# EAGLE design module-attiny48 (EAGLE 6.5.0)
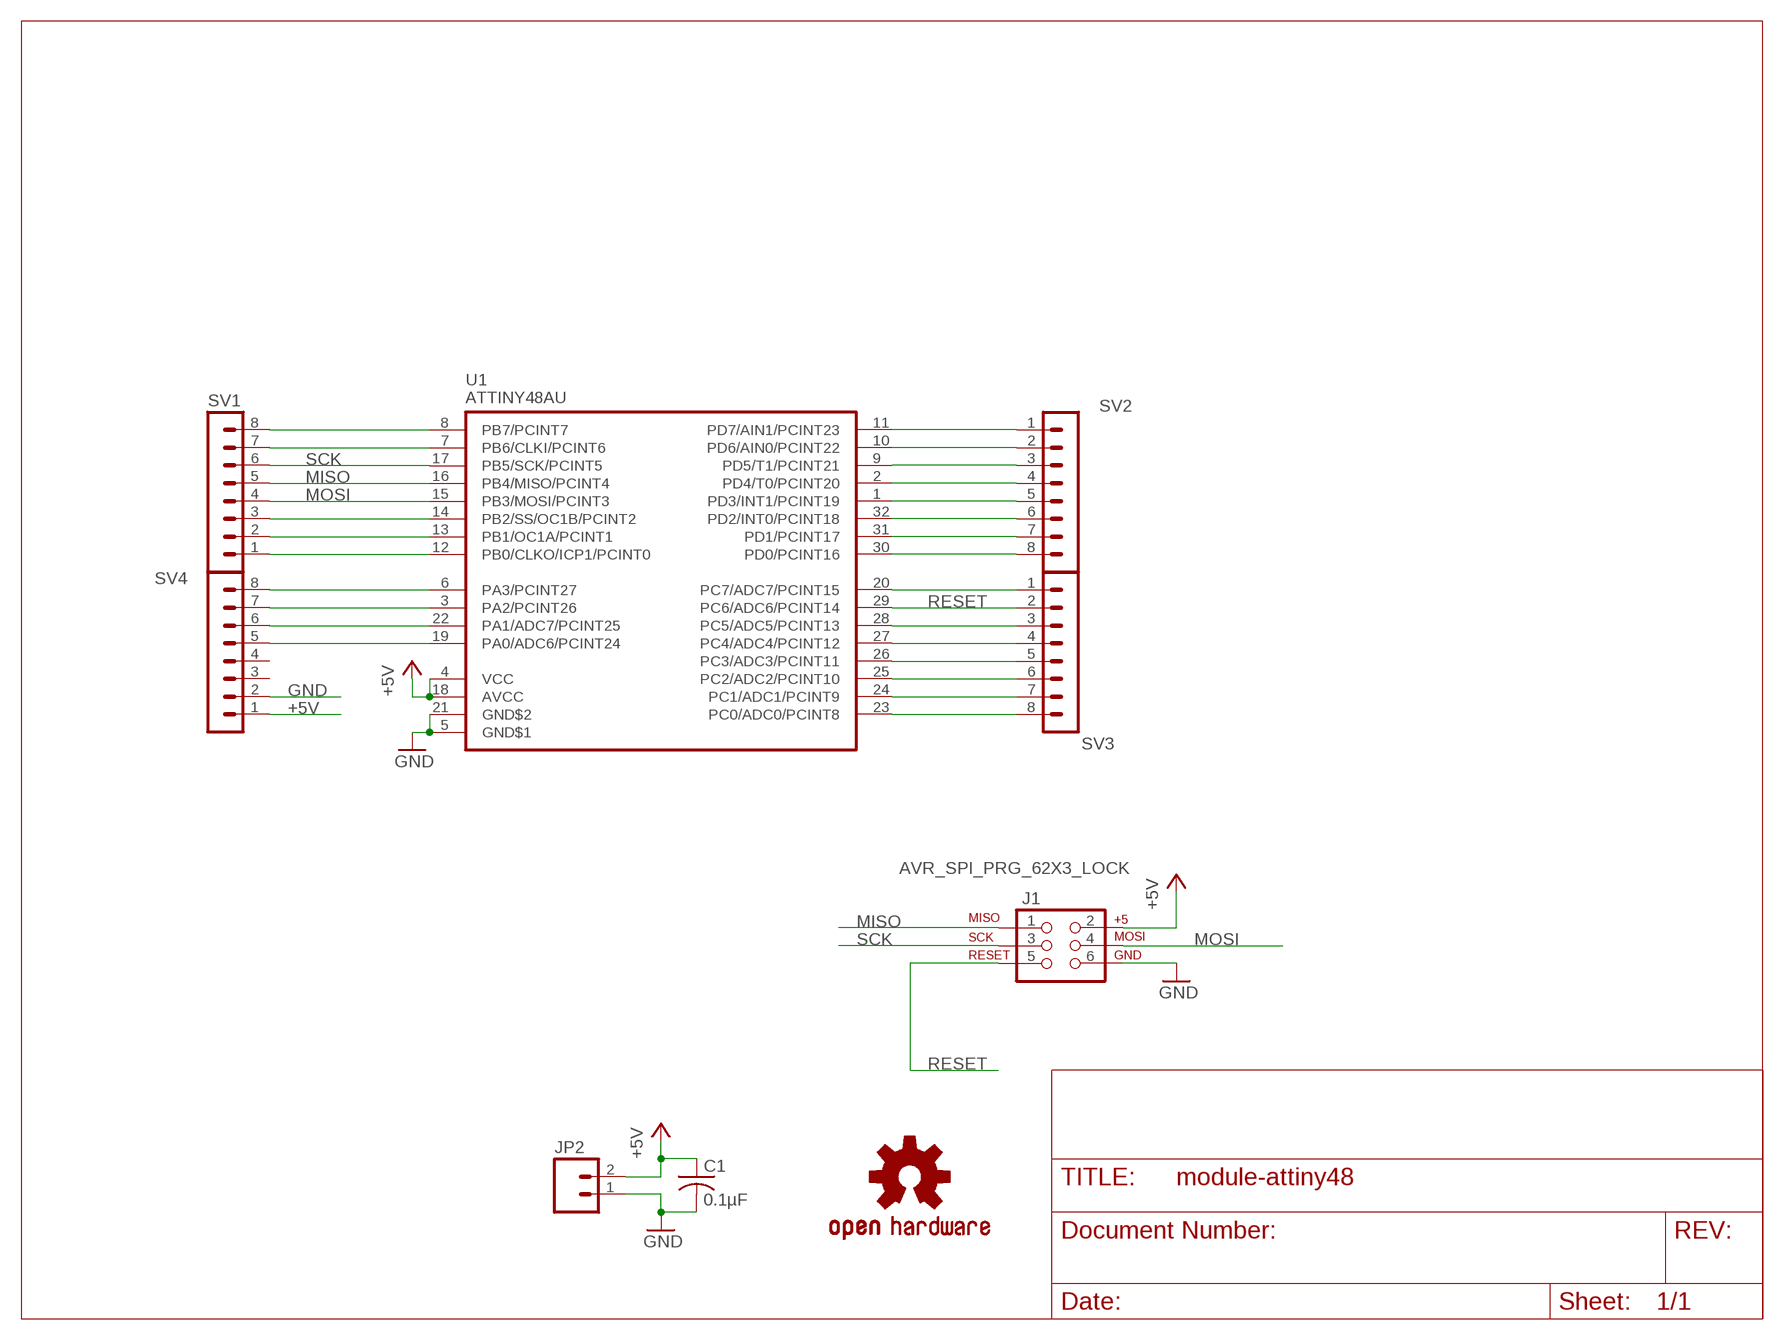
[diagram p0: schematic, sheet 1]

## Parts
C1  0.1µF  C-USC0805  [C0805]
J1  AVR_SPI_PRG_62X3_LOCK  [2X3_LOCK]
JP2  M02LOCK_LONGPADS  [1X02_LOCK_LONGPADS]
SV1  MA08-1  [MA08-1]
SV2  MA08-1  [MA08-1]
SV3  MA08-1  [MA08-1]
SV4  MA08-1  [MA08-1]
U1  ATTINY48AU  [TQFP32-08]
U$1  OSHW-LOGOS  [OSHW-LOGO-S]

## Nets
+5V: C1.1 J1.2 JP2.2 SV4.1 U1.4(VCC) U1.18(AVCC)
GND: C1.2 J1.6 JP2.1 SV4.2 U1.5(GND$1) U1.21(GND$2)
MISO: J1.1 SV1.5 U1.16(PB4/MISO/PCINT4)
MOSI: J1.4 SV1.4 U1.15(PB3/MOSI/PCINT3)
N$3: SV1.1 U1.12(PB0/CLKO/ICP1/PCINT0)
N$4: SV1.2 U1.13(PB1/OC1A/PCINT1)
N$5: SV1.3 U1.14(PB2/SS/OC1B/PCINT2)
N$6: SV3.1 U1.20(PC7/ADC7/PCINT15)
N$7: SV3.3 U1.28(PC5/ADC5/PCINT13)
N$8: SV3.4 U1.27(PC4/ADC4/PCINT12)
N$9: SV1.7 U1.7(PB6/CLKI/PCINT6)
N$10: SV1.8 U1.8(PB7/PCINT7)
N$11: SV2.1 U1.11(PD7/AIN1/PCINT23)
N$12: SV2.2 U1.10(PD6/AIN0/PCINT22)
N$13: SV3.5 U1.26(PC3/ADC3/PCINT11)
N$14: SV3.6 U1.25(PC2/ADC2/PCINT10)
N$15: SV3.7 U1.24(PC1/ADC1/PCINT9)
N$16: SV3.8 U1.23(PC0/ADC0/PCINT8)
N$17: SV2.3 U1.9(PD5/T1/PCINT21)
N$18: SV2.4 U1.2(PD4/T0/PCINT20)
N$19: SV2.5 U1.1(PD3/INT1/PCINT19)
N$20: SV2.6 U1.32(PD2/INT0/PCINT18)
N$21: SV2.7 U1.31(PD1/PCINT17)
N$22: SV2.8 U1.30(PD0/PCINT16)
N$23: SV4.8 U1.6(PA3/PCINT27)
N$24: SV4.7 U1.3(PA2/PCINT26)
N$25: SV4.6 U1.22(PA1/ADC7/PCINT25)
N$26: SV4.5 U1.19(PA0/ADC6/PCINT24)
RESET: J1.5 SV3.2 U1.29(PC6/ADC6/PCINT14)
SCK: J1.3 SV1.6 U1.17(PB5/SCK/PCINT5)
Unconnected: SV4.3 SV4.4

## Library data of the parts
C1 = rcl:C-US: CAPACITOR, American symbol
J1 = SparkFun:AVR_SPI_PRG_6: AVR ISP 6 Pin This is the reduced ISP connector for AVR programming. Common on Arduino. This footprint will take up less PCB space and can be used with a 10-pin to 6-pin adapter such as SKU: BOB-08508
JP2 = SparkFun:M02: Header 2
SV1-SV4 = con-lstb:MA08-1: PIN HEADER; OC_FARNELL: unknown; OC_NEWARK: unknown
U1 = attiny48:ATTINY48: Atmel ATtiny48-AU in 32-pin TQFP package
U$1 = SparkFun:OSHW-LOGO: Open Source Hardware Logo This logo indicates the piece of hardware it is found on incorporates a OSHW license and/or adheres to the definition of open source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

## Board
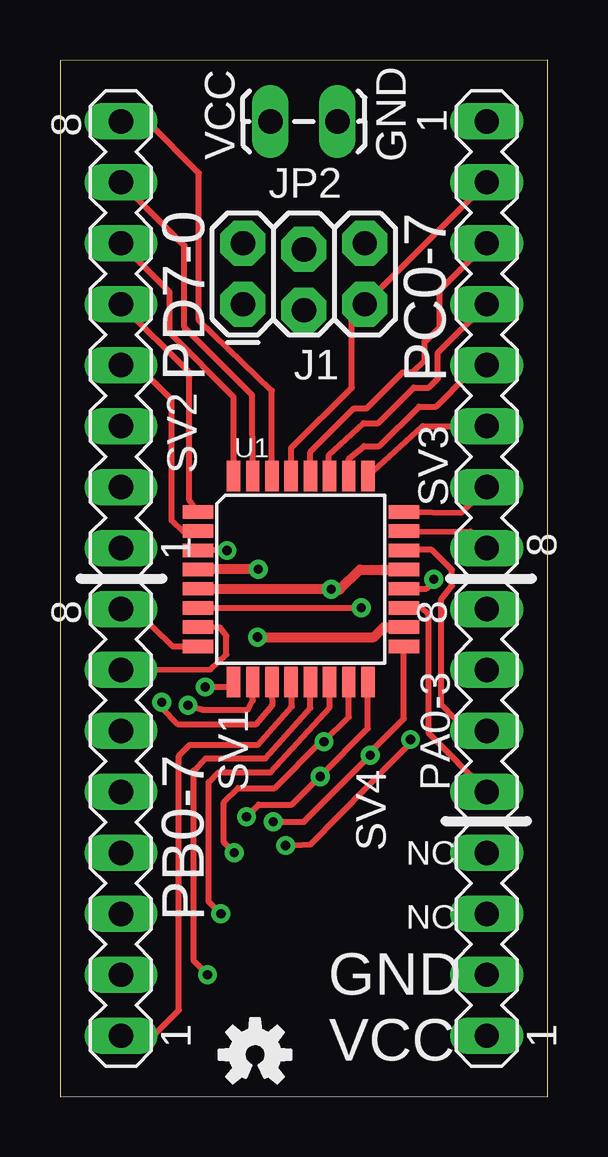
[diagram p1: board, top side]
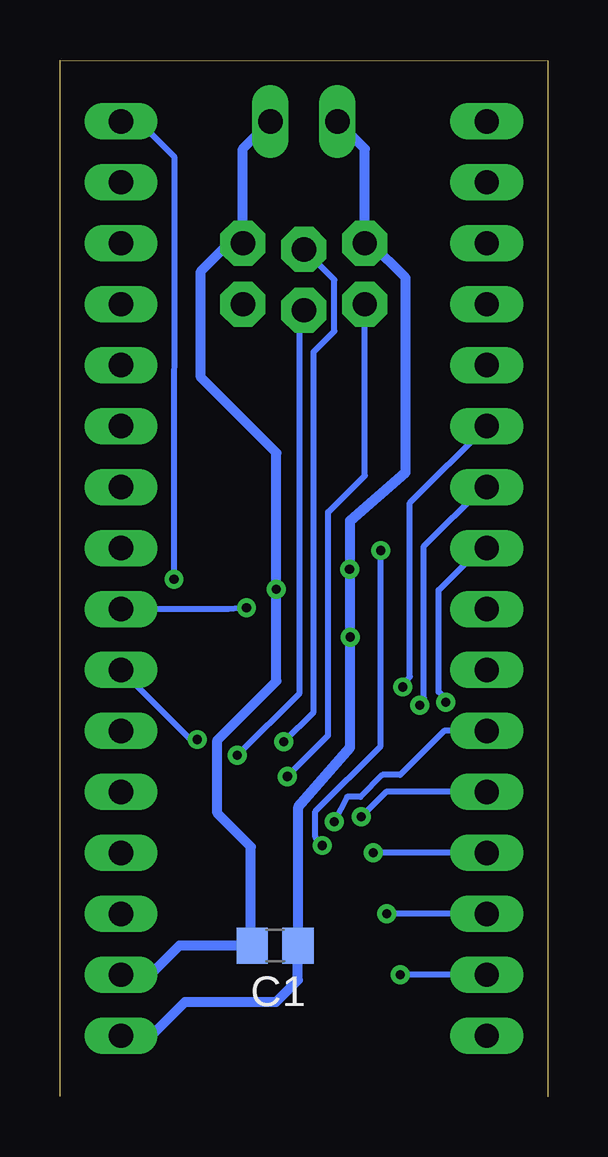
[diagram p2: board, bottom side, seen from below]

Size 20.32 x 43.2 mm. Coordinates in mm from the lower left corner, seen from the top.
Outline: 20.32,0.03 20.32,43.2 0,43.17 0,0
Copper layers (1*16): Top 0.035mm / dielectric 1.5mm / Bottom 0.035mm
Design rules "default": minimum track width 10mil, minimum drill 24mil, track to track 8mil, track to pad 8mil, pad to pad 8mil, via to via 8mil, smd to smd 8mil, copper to edge 40mil, drill to drill 8mil, minimum pad ring 10mil, minimum via ring 8mil, stop-mask expansion 4mil, vias tented up to drill 0mil, thermal gap 10mil

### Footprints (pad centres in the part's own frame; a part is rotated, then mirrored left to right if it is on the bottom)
C0805 = smd 1.3 x 1.5: 1 -0.95,0; 2 0.95,0
2X3_LOCK = drill 1.016 pad 1.88 octagon: 1 0,0; 2 0,2.54; 3 2.54,-0.254; 4 2.54,2.286; 5 5.08,0; 6 5.08,2.54
1X02_LOCK_LONGPADS = drill 1.016 long: 1 -0.127,0; 2 2.667,0
MA08-1 = drill 1.016 long: 1 -8.89,0; 2 -6.35,0; 3 -3.81,0; 4 -1.27,0; 5 1.27,0; 6 3.81,0; 7 6.35,0; 8 8.89,0
TQFP32-08 = smd 1.27 x 0.559: 1 -4.293,2.8; 2 -4.293,2; 3 -4.293,1.2; 4 -4.293,0.4; 5 -4.293,-0.4; 6 -4.293,-1.2; 7 -4.293,-2; 8 -4.293,-2.8; 17 4.293,-2.8; 18 4.293,-2; 19 4.293,-1.2; 20 4.293,-0.4; 21 4.293,0.4; 22 4.293,1.2; 23 4.293,2; 24 4.293,2.8 | smd 0.559 x 1.27: 9 -2.8,-4.293; 10 -2,-4.293; 11 -1.2,-4.293; 12 -0.4,-4.293; 13 0.4,-4.293; 14 1.2,-4.293; 15 2,-4.293; 16 2.8,-4.293; 25 2.8,4.293; 26 2,4.293; 27 1.2,4.293; 28 0.4,4.293; 29 -0.4,4.293; 30 -1.2,4.293; 31 -2,4.293; 32 -2.8,4.293

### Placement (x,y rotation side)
C1  11.35,6.3 180 bottom
J1  7.62,33.02 0 top
JP2  11.43,40.64 180 top
SV1  2.54,11.43 90 top
SV2  2.54,31.75 90 top
SV3  17.78,31.75 270 top
SV4  17.78,11.43 90 top
U1  10.03,21.56 0 top
U$1  8.13,1.75 0 top

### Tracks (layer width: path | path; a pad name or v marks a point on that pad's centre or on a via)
+5V  (via drill 0.38)
  Top 0.406: U1.18 13.49,19.57 13.08,19.15 v8.23,19.15 | v8.26,21.97 U1.4
  Bottom 0.406: 8.23,22 v8.23,19.15 8.23,14.55 10.39,12.09 10.39,6.31 C1.1 10.4,4.86 11.33,3.94 15.11,3.94 16.56,2.49 17.73,2.49 SV4.1 | JP2.2 7.62,39.5 J1.2 7.37,35.56 5.92,34.11 5.92,26.01 8.23,24 8.23,22 | 8.23,22 v8.26,21.97
GND  (via drill 0.38)
  Top 0.406: U1.5 5.77,21.14 v11.31,21.14 11.66,21.14 12.49,21.96 U1.21
  Bottom 0.406: JP2.1 12.7,39.5 J1.6 13.28,35.56 14.45,34.39 14.45,29.97 11.31,26.83 v11.31,21.14 11.31,17.32 13.77,14.86 13.77,11.81 12.37,10.41 12.37,6.37 C1.2 15.34,6.3 16.51,5.13 17.73,5.13 SV4.2
MISO  (via drill 0.38)
  Top 0.254: v7.77,11.66 8.28,12.17 9.66,12.17 v10.84,13.35 12.83,15.34 U1.16
  Bottom 0.254: v7.77,11.66 6.73,12.7 SV1.5 | J1.1 7.62,25.88 9.14,24.36 9.14,15.05 v10.84,13.35
MOSI  (via drill 0.38)
  Top 0.254: 12.04,17.23 U1.15 12.03,15.82 v11,14.78 10.87,14.78 8.94,12.85 7.42,12.85 6.83,12.27 6.83,10.59 v7.26,10.16
  Bottom 0.254: SV1.4 v7.26,10.16 | J1.4 8.89,34.04 8.89,31.9 9.75,31.04 9.75,16.03 v11,14.78
N$1  (via drill 0.38)
  other vias: 10.85,13.34
N$3
  Top 0.254: U1.12 9.66,16.26 8.23,14.66 5.41,14.66 4.95,14.2 4.95,3.61 3.89,2.54 SV1.1
N$4  (via drill 0.38)
  Top 0.254: U1.13 10.43,16.2 8.56,14.1 6.07,14.1 5.56,13.59 5.56,5.66 v6.15,5.08
  Bottom 0.254: SV1.2 v6.15,5.08
N$5  (via drill 0.38)
  Top 0.254: U1.14 11.23,16.24 8.76,13.51 6.6,13.51 6.2,13.11 6.2,8.13 v6.71,7.62
  Bottom 0.254: SV1.3 v6.71,7.62
N$6  (via drill 0.38)
  Top 0.254: U1.20 15.27,21.16 v15.57,21.57
  Bottom 0.254: v15.57,21.57 15.54,39.14 17.04,40.64 SV3.1
N$7
  Top 0.254: U1.28 10.43,26.87 12.24,28.68 12.78,28.68 14.28,30.18 14.71,30.18 15.19,30.66 15.19,31.45 15.82,32.08 15.82,33.6 SV3.3
N$8
  Top 0.254: U1.27 11.21,26.73 12.65,28.07 13.26,28.07 14.73,29.54 15.37,29.54 15.75,29.92 15.75,30.99 SV3.4
N$9
  Top 0.254: U1.7 6.67,19.54 6.93,19.2 6.93,18.41 6.27,17.8 SV1.7
N$10
  Top 0.254: U1.8 4.71,18.77 3.12,20.32 SV1.8
N$11  (via drill 0.38)
  Top 0.254: U1.11 8.86,16.33 8.18,15.52 4.9,15.52 4.24,16.2 v4.24,16.43
  Bottom 0.254: SV2.1 2.79,22.86 4.55,21.11 4.55,16.87 4.24,16.56 v4.24,16.43
N$12  (via drill 0.38)
  Top 0.254: U1.10 8.03,16.52 7.82,16.13 5.94,16.13 v5.33,16.31
  Bottom 0.254: SV2.2 2.69,25.4 5.16,22.94 5.16,16.61 v5.33,16.31
N$13
  Top 0.254: U1.26 12.03,26.59 12.68,27.1 13.31,27.1 14.96,28.75 15.67,28.75 16.99,30.07 17.37,30.07 SV3.5
N$14
  Top 0.254: U1.25 15.12,27.94 SV3.6
N$15
  Top 0.254: U1.24 16.72,24.34 SV3.7
N$16
  Top 0.254: U1.23 17.1,23.54 SV3.8
N$17  (via drill 0.38)
  Top 0.254: U1.9 7.18,17.07 v6.04,17.07
  Bottom 0.254: SV2.3 5.74,24.74 5.74,17.5 v6.04,17.07
N$18
  Top 0.254: U1.2 5.14,23.54 4.65,24 4.65,29.03 3.23,30.48 SV2.4
N$19
  Top 0.254: U1.1 5.38,24.87 5.38,30.18 SV2.5
N$20
  Top 0.254: U1.32 7.23,29.14 4.57,31.83 4.57,33.53 SV2.6
N$21
  Top 0.254: U1.31 8.01,29.23 5.18,32.05 5.18,35.46 SV2.7
N$22
  Top 0.254: U1.30 8.83,29.42 5.79,32.36 5.79,38.48 3.63,40.64 SV2.8
N$23  (via drill 0.38)
  Top 0.254: U1.6 10.62,20.36 v12.55,20.37
  Bottom 0.254: v12.55,20.37 13.31,20.32 SV4.8
N$24  (via drill 0.38)
  Top 0.254: U1.3 v6.95,22.77 v6.96,22.76 | v9.4,10.46 10.44,10.52 14.02,14.15 14.61,14.76 v14.61,14.88
  Bottom 0.254: v6.96,22.76 6.96,14.61 9.68,11.89 9.68,10.82 v9.4,10.46 | v14.61,14.88 14.91,14.91 SV4.7
N$25
  Top 0.254: U1.22 14.46,22.78 15.49,22.78 16.33,21.95 16.33,21.29 15.88,20.73 15.88,16.36 16.94,15.24 SV4.6
N$26
  Top 0.254: U1.19 15.07,20.36 15.37,20.09 15.37,15.14 SV4.5
RESET
  Top 0.254: U1.29 9.63,27.03 12.17,29.54 12.17,32.49 J1.5 SV3.2
SCK  (via drill 0.38)
  Top 0.254: U1.17 14.33,15.75 12.93,14.35 v12.93,14.22 10.16,11.46 v8.89,11.46
  Bottom 0.254: v8.89,11.46 8.36,12.5 7.8,12.5 6.88,13.41 6.15,13.41 4.32,15.24 SV1.6 | J1.3 10.34,32.59 10.34,16.82 v12.93,14.22

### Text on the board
tNames: VCC | GND | PD7-0 | PC0-7 | PA0-3 | NC | PB0-7 | NC | GND | VCC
